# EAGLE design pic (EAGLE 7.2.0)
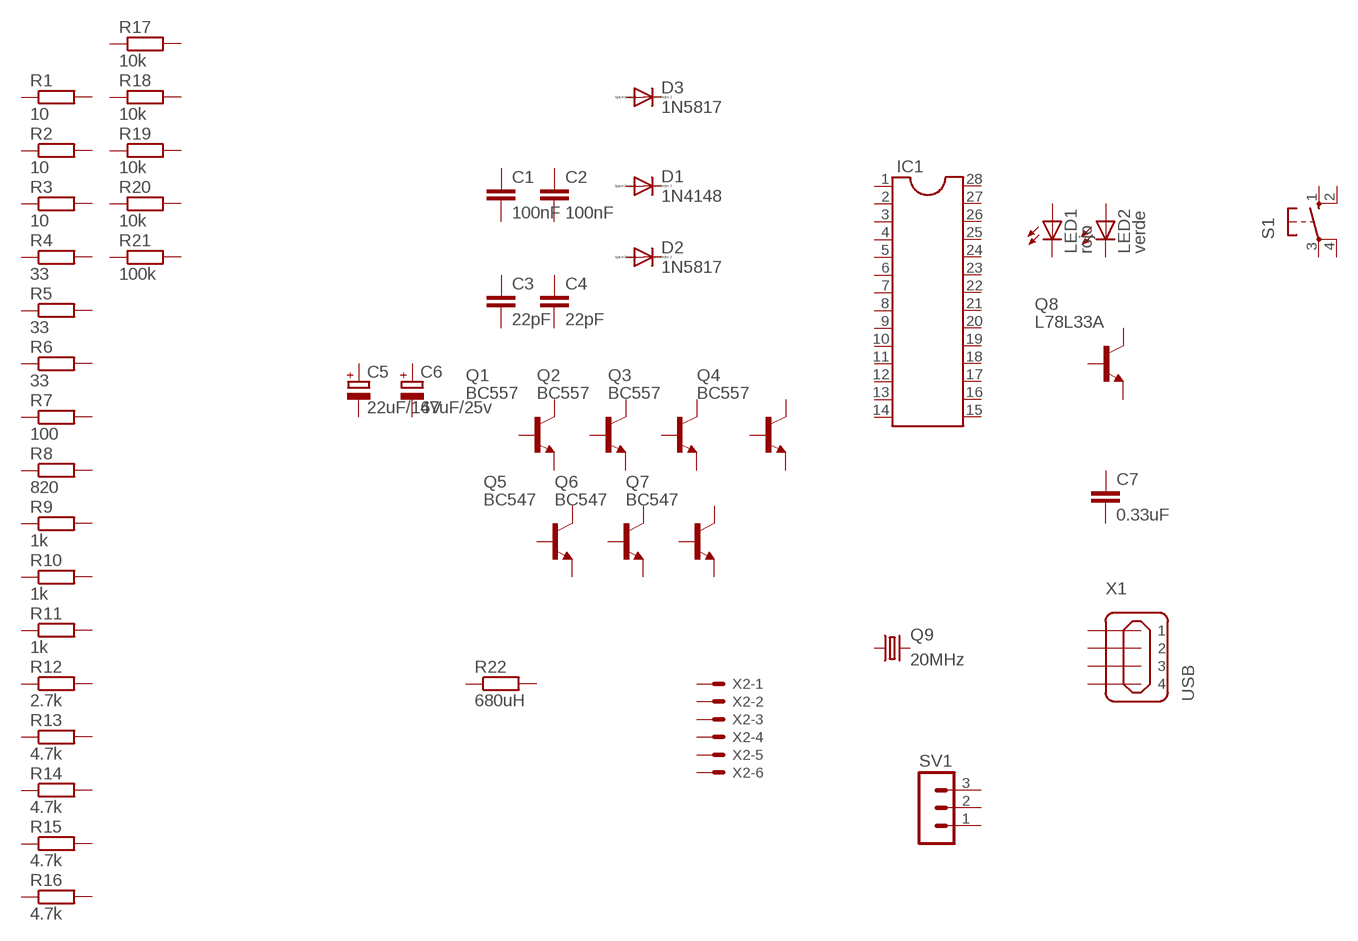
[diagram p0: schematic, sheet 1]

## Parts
C1  100nF  C-EU025-030X050  [C025-030X050]
C2  100nF  C-EU025-030X050  [C025-030X050]
C3  22pF  C-EU050-024X044  [C050-024X044]
C4  22pF  C-EU050-024X044  [C050-024X044]
C5  22uF/16V  CPOL-EUE2-5  [E2-5]
C6  47uF/25v  CPOL-EUE2-5  [E2-5]
C7  0.33uF  C-EU050-024X044  [C050-024X044]
D1  1N4148  1N4148DO35-7  [DO35-7]
D2  1N5817  1N4148DO35-7  [DO35-7]
D3  1N5817  1N4148DO35-7  [DO35-7]
IC1  DIL28-3  [DIL28-3]
LED1  rojo  LED3MM  [LED3MM]
LED2  verde  LED3MM  [LED3MM]
Q1  BC557  BCX59SMD  [TO92-EBC]
Q2  BC557  BCX59SMD  [TO92-EBC]
Q3  BC557  BCX59SMD  [TO92-EBC]
Q4  BC557  BCX59SMD  [TO92-EBC]
Q5  BC547  BCX59SMD  [TO92-EBC]
Q6  BC547  BCX59SMD  [TO92-EBC]
Q7  BC547  BCX59SMD  [TO92-EBC]
Q8  L78L33A  BC449  [TO92-EBC]
Q9  20MHz  CRYSTALHC49S  [HC49/S]
R1  10  R-EU_0207/7  [0207/7]
R2  10  R-EU_0207/7  [0207/7]
R3  10  R-EU_0207/7  [0207/7]
R4  33  R-EU_0207/7  [0207/7]
R5  33  R-EU_0207/7  [0207/7]
R6  33  R-EU_0207/7  [0207/7]
R7  100  R-EU_0207/7  [0207/7]
R8  820  R-EU_0207/7  [0207/7]
R9  1k  R-EU_0207/7  [0207/7]
R10  1k  R-EU_0207/7  [0207/7]
R11  1k  R-EU_0207/7  [0207/7]
R12  2.7k  R-EU_0207/7  [0207/7]
R13  4.7k  R-EU_0207/7  [0207/7]
R14  4.7k  R-EU_0207/7  [0207/7]
R15  4.7k  R-EU_0207/7  [0207/7]
R16  4.7k  R-EU_0207/7  [0207/7]
R17  10k  R-EU_0207/7  [0207/7]
R18  10k  R-EU_0207/7  [0207/7]
R19  10k  R-EU_0207/7  [0207/7]
R20  10k  R-EU_0207/7  [0207/7]
R21  100k  R-EU_0207/7  [0207/7]
R22  680uH  R-EU_0207/10  [0207/10]
S1  10-XX  [B3F-10XX]
SV1  MA03-1  [MA03-1]
X1  USB  MINI-USB_SHIELD4P-85-32004-00X  [85-32004-00X]
X2  22-23-2061  [22-23-2061]
Unconnected: C1.1 C1.2 C2.1 C2.2 C3.1 C3.2 C4.1 C4.2 C5.+ C5.- C6.+ C6.- C7.1 C7.2 D1.A D1.C D2.A D2.C D3.A D3.C IC1.1 IC1.2 IC1.3 IC1.4 IC1.5 IC1.6 IC1.7 IC1.8 IC1.9 IC1.10 IC1.11 IC1.12 IC1.13 IC1.14 IC1.15 IC1.16 IC1.17 IC1.18 IC1.19 IC1.20 IC1.21 IC1.22 IC1.23 IC1.24 IC1.25 IC1.26 IC1.27 IC1.28 LED1.A LED1.K(C) LED2.A LED2.K(C) Q1.B Q1.C Q1.E Q2.B Q2.C Q2.E Q3.B Q3.C Q3.E Q4.B Q4.C Q4.E Q5.B Q5.C Q5.E Q6.B Q6.C Q6.E Q7.B Q7.C Q7.E Q8.B Q8.C Q8.E Q9.1 Q9.2 R1.1 R1.2 R2.1 R2.2 R3.1 R3.2 R4.1 R4.2 R5.1 R5.2 R6.1 R6.2 R7.1 R7.2 R8.1 R8.2 R9.1 R9.2 R10.1 R10.2 R11.1 R11.2 R12.1 R12.2 R13.1 R13.2 R14.1 R14.2 R15.1 R15.2 R16.1 R16.2 R17.1 R17.2 R18.1 R18.2 R19.1 R19.2 R20.1 R20.2 R21.1 R21.2 R22.1 R22.2 S1.1(S) S1.2(S1) S1.3(P) S1.4(P1) SV1.1 SV1.2 SV1.3 X1.1 X1.2 X1.3 X1.4 X1.M1(S1) X1.M2(S2) X2.1 X2.2 X2.3 X2.4 X2.5 X2.6

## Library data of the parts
C1-C4 C7 = rcl:C-EU: CAPACITOR, European symbol
C5 C6 = rcl:CPOL-EU: POLARIZED CAPACITOR, European symbol
D1-D3 = diode:1N4148: DIODE
IC1 = ic-package:DIL28: Dual In Line
LED1 LED2 = led:LED: LED
Q1-Q7 = transistor-npn:BCX59*: NPN Transistor
Q8 = transistor-npn:BC449*: NPN Transistor
Q9 = crystal:CRYSTAL: CRYSTAL; OC_FARNELL: 1667008; OC_NEWARK: unknown
R1-R22 = rcl:R-EU_: RESISTOR, European symbol
S1 = switch-omron:10-XX: OMRON SWITCH; MPN: B3F-1000; OC_FARNELL: 176432; OC_NEWARK: 36M3542
SV1 = con-lstb:MA03-1: PIN HEADER; OC_FARNELL: unknown; OC_NEWARK: unknown
X1 = con-cypressindustries:MINI-USB_SHIELD4P-: MINI USB 4 Pol. Source: www.cypressindustries.com; OC_FARNELL: unknown; OC_NEWARK: unknown
X2 = con-molex:22-23-2061: .100" (2.54mm) Center Header - 6 Pin; MF: MOLEX; MPN: 22-23-2061; OC_FARNELL: 1462922; OC_NEWARK: 27C1933

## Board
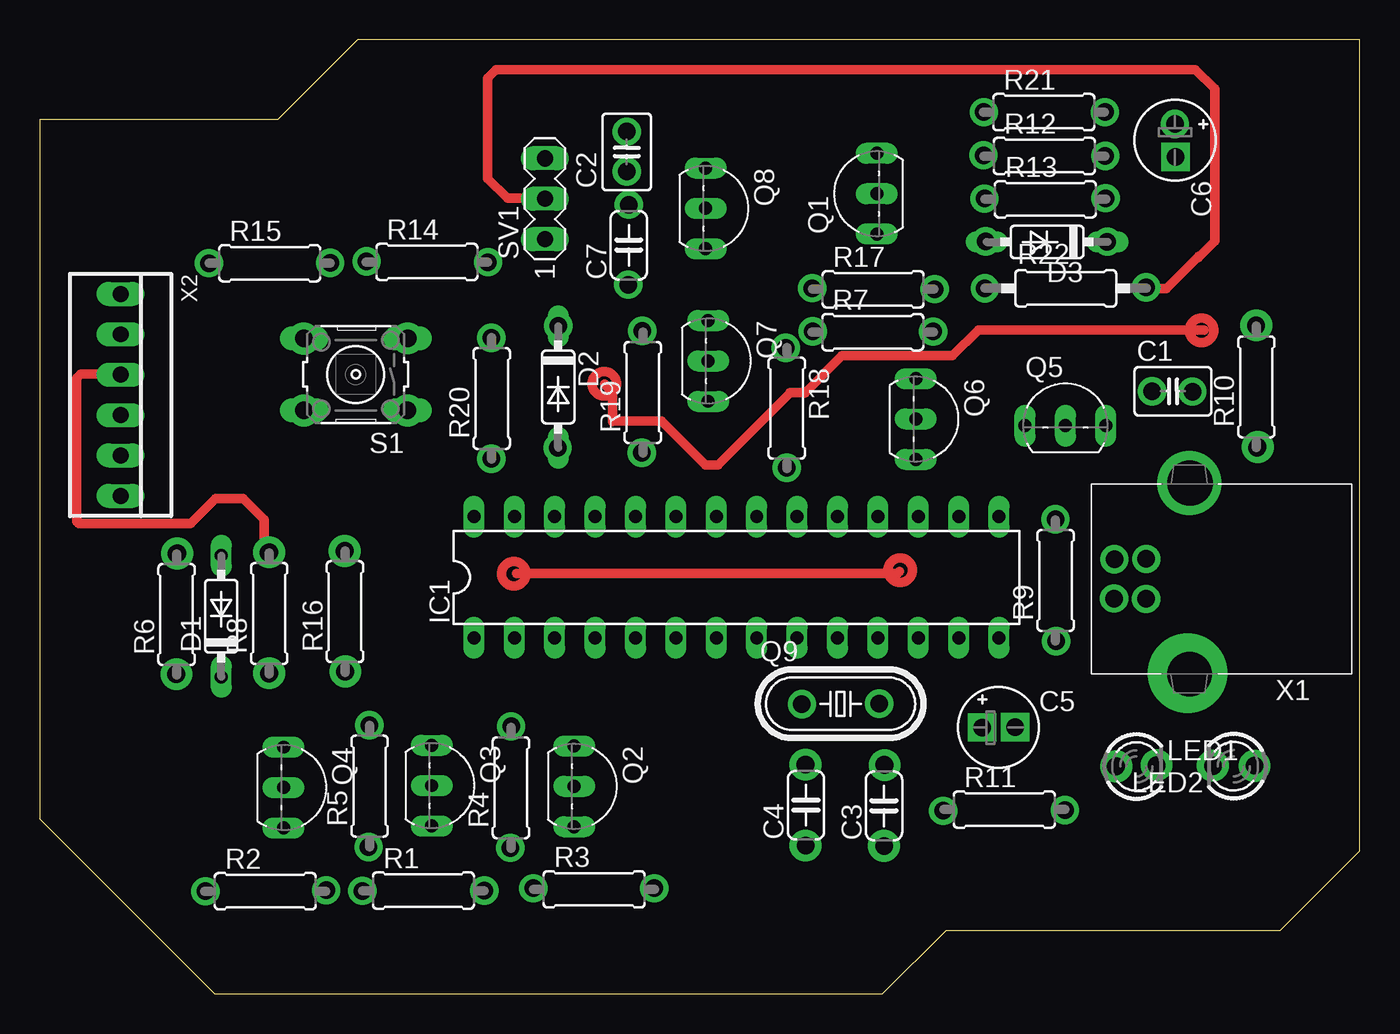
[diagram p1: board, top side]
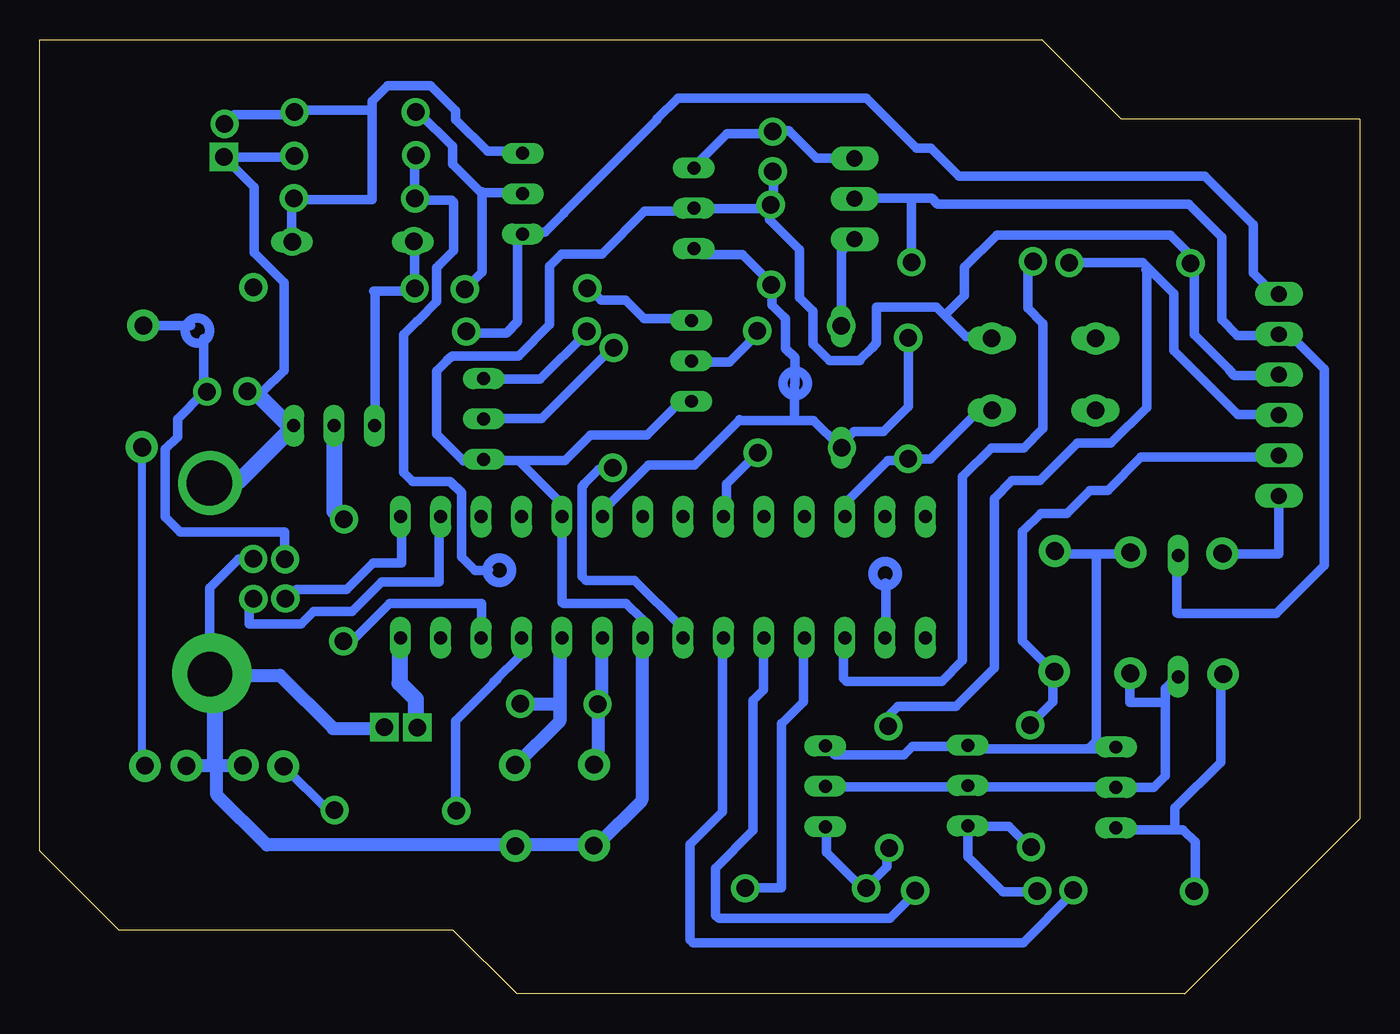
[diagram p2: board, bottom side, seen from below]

Size 83 x 60 mm. Coordinates in mm from the lower left corner, seen from the top.
Outline: 83,60 20,60 15,55 0,55 0,30 0,11 11,0 53,0 57,4 78,4 83,9 83,60
Copper layers (1*16): Top 0.035mm / dielectric 1.5mm / Bottom 0.035mm
Design rules "default": minimum track width 10mil, minimum drill 24mil, track to track 8mil, track to pad 8mil, pad to pad 8mil, via to via 8mil, smd to smd 8mil, copper to edge 40mil, drill to drill 8mil, minimum pad ring 10mil, minimum via ring 8mil, stop-mask expansion 4mil, vias tented up to drill 0mil, thermal gap 10mil

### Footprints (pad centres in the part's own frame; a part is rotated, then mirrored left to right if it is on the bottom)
C025-030X050 = drill 0.813 octagon: 1 -1.27,0; 2 1.27,0
C050-024X044 = drill 0.813 octagon: 1 -2.54,0; 2 2.54,0
E2-5 = drill 0.813 pad 1.27: + -1.016,0 | drill 0.813 pad 1.27 octagon: - 1.016,0
DO35-7 = drill 0.813 long: A 3.81,0; C -3.81,0
DIL28-3 = drill 0.813 long: 1 -16.51,-3.81; 2 -13.97,-3.81; 3 -11.43,-3.81; 4 -8.89,-3.81; 5 -6.35,-3.81; 6 -3.81,-3.81; 7 -1.27,-3.81; 8 1.27,-3.81; 9 3.81,-3.81; 10 6.35,-3.81; 11 8.89,-3.81; 12 11.43,-3.81; 13 13.97,-3.81; 14 16.51,-3.81; 15 16.51,3.81; 16 13.97,3.81; 17 11.43,3.81; 18 8.89,3.81; 19 6.35,3.81; 20 3.81,3.81; 21 1.27,3.81; 22 -1.27,3.81; 23 -3.81,3.81; 24 -6.35,3.81; 25 -8.89,3.81; 26 -11.43,3.81; 27 -13.97,3.81; 28 -16.51,3.81
LED3MM = drill 0.813 octagon: A -1.27,0; K 1.27,0
TO92-EBC = drill 0.813 long: B 0,-1.27; C -2.54,-1.27; E 2.54,-1.27
HC49/S = drill 0.813: 1 -2.413,0; 2 2.413,0
0207/7 = drill 0.813 octagon: 1 -3.81,0; 2 3.81,0
0207/10 = drill 0.813 octagon: 1 -5.08,0; 2 5.08,0
B3F-10XX = drill 1.016 long: 1 -3.251,2.261; 2 3.251,2.261; 3 -3.251,-2.261; 4 3.251,-2.261
MA03-1 = drill 1.016 long: 1 -2.54,0; 2 0,0; 3 2.54,0
85-32004-00X = drill 0.92 pad 1.27: 1 4.71,-1.25; 2 4.71,1.25; 3 2.71,1.25; 4 2.71,-1.25 | drill 2.3 pad 3: M1 0,6.02; M2 0,-6.02
22-23-2061 = drill 1 long: 1 -6.35,0; 2 -3.81,0; 3 -1.27,0; 4 1.27,0; 5 3.81,0; 6 6.35,0

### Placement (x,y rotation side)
C1  71.25,37.89 0 top
C2  36.91,52.95 90 top
C3  53.09,11.82 90 top
C4  48.17,11.86 90 top
C5  60.28,16.75 0 top
C6  71.39,53.68 270 top
C7  37.04,47.08 90 top
D1  11.41,23.75 90 top
D2  32.6,38.16 270 top
D3  63.34,47.29 180 top
IC1  43.81,26.2 0 top
LED1  68.95,14.3 0 top
LED2  75.08,14.31 180 top
Q1  51.37,50.32 90 top
Q2  34.88,13.05 270 top
Q3  25.91,13.1 270 top
Q4  16.6,12.97 270 top
Q5  64.5,37 0 top
Q6  56.35,36.15 270 top
Q7  43.29,39.8 270 top
Q8  43.14,49.4 270 top
Q9  50.35,18.24 0 top
R1  24.12,6.49 0 top
R2  14.18,6.46 0 top
R3  34.86,6.57 0 top
R4  29.63,12.96 90 top
R5  20.74,13.06 90 top
R6  8.6,23.85 90 top
R7  52.38,41.61 0 top
R8  14.43,23.92 90 top
R9  63.87,26 90 top
R10  76.5,38.17 90 top
R11  60.65,11.59 0 top
R12  63.16,52.69 0 top
R13  63.23,49.97 0 top
R14  24.34,46.03 0 top
R15  14.46,45.95 0 top
R16  19.19,24.04 90 top
R17  52.4,44.31 0 top
R18  46.97,36.84 270 top
R19  37.92,37.82 90 top
R20  28.42,37.45 90 top
R21  63.13,55.45 0 top
R22  64.51,44.37 0 top
S1  19.88,38.95 180 top
SV1  31.76,50 90 top
X1  72.28,26.09 180 top
X2  5.08,37.66 270 top

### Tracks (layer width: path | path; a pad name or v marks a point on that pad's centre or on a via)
N$1  (via drill 1.1 pad 1.78)
  other vias: 67.58,27.32
N$2  (via drill 1.1 pad 1.78)
  other vias: 69.58,27.35
N$3  (via drill 1.1 pad 1.78)
  other vias: 67.55,24.86
N$4  (via drill 1.1 pad 1.78)
  other vias: 69.56,24.84
N$5  (via drill 2.8 pad 3.81)
  other vias: 72.35,32.1
N$6  (via drill 2.8 pad 4)
  other vias: 72.3,20.11
N$7  (via drill 2.8 pad 4)
  other vias: 72.29,32.12
N$8
  Bottom 0.5: 76.59,34.34 76.59,14.53 76.42,14.36
N$9
  Bottom 0.61: 69.69,27.34 70.5,27.34 72.33,25.51 72.33,21.51 72.35,21.49
N$10
  Bottom 0.813: 72.15,20.02 67.9,20.02 64.56,16.69 61.42,16.69 61.33,16.79
N$11
  Bottom 0.813: 70.38,14.34 73.64,14.34 73.66,14.31
N$12
  Bottom 0.813: 72.08,14.36 72.08,19.99 72.12,20.04
N$13
  Bottom 0.5: 59.26,16.8 59.26,18.51 60.48,19.73 60.48,22.21 60.42,22.26
N$14
  Bottom 0.61: 64.46,11.53 64.86,11.53 67.59,14.25
N$15
  Bottom 0.61: 67.59,27.34 67.59,29.04 74.16,29.04 75.1,29.98 75.1,34.26 74.34,35.02 74.34,36.15 72.69,37.8 72.69,41.21
N$16
  Bottom 0.61: 76.42,42.09 76.38,42.04 73.51,42.04
N$17
  Bottom 0.61: 56.85,11.54 56.85,17.18 54.24,19.79
N$18
  Bottom 0.61: 47.61,22.31 47.61,18.66 47.88,18.4 47.88,14.7 48.11,14.46
N$19
  Bottom 0.61: 50.15,22.4 50.15,17.24 53.05,14.34
N$20
  Bottom 0.61: 52.7,18.19 50.34,18.19 50.31,18.21
N$21  (via drill 1.1 pad 1.78)
  other vias: 52.77,18.25
N$22  (via drill 1.1 pad 1.78)
  other vias: 47.92,18.21
N$23  (via drill 1.1 pad 1.78)
  other vias: 48.16,14.41
N$24  (via drill 1.1 pad 1.78)
  other vias: 53.11,14.4
N$25  (via drill 1.1 pad 1.78)
  other vias: 48.16,9.34
N$26  (via drill 1.1 pad 1.78)
  other vias: 53.11,9.3
N$27
  Bottom 0.61: 52.73,22.3 52.74,22.31
N$28
  Bottom 0.61: 52.71,22.3 52.71,21.34 54.45,19.6
N$29
  Bottom 0.61: 48.19,9.29 52.95,9.29 52.98,9.31 68.69,9.31 71.95,12.57 71.95,14.3 72.04,14.39
N$30
  Bottom 0.61: 61.92,35.81 61.92,44.11 62,44.19 59.62,44.19 59.42,44.39 59.42,47.25
N$31
  Bottom 0.61: 63.92,22.21 63.31,22.21 60.99,24.54 55.23,24.54 55.21,24.52 | 55.21,22.44 55.21,24.52 | 55.21,24.52 55.21,24.54
N$32
  Bottom 0.61: 57.89,29.98 57.89,25.89 61.51,25.89 63.36,24.04 65.78,24.04 66.56,23.25 69.8,23.25 69.83,23.27 69.83,24.52 69.6,24.75
N$33
  Bottom 0.61: 60.24,29.89 60.24,27.1 62.02,27.1 63.7,25.43 66.85,25.43 67.44,24.84
N$34
  Bottom 0.61: 64.58,35.54 64.58,30.56 63.92,29.91
N$35
  Bottom 0.61: 72.24,32.27 70.44,32.27 67.12,35.59
N$36
  Bottom 0.61: 69.85,37.77 69.14,37.77 67.1,35.74
N$37
  Bottom 1.016: 72.01,32.24 70.46,32.24 67.25,35.45 67.25,35.65 69.41,37.81
N$38
  Bottom 1.016: 64.49,35.49 64.49,30.36 63.92,29.8
N$39
  Bottom 1.016: 60.38,22.23 60.38,19.55 59.36,18.54 59.36,17.06 59.21,16.91
N$40
  Bottom 0.61: 67.15,47.09 67.15,49.83 67.06,49.91
N$41
  Bottom 0.61: 59.42,49.99 59.42,52.49 59.35,52.56
N$42
  Bottom 0.61: 71.4,52.61 67.16,52.61 67.11,52.56
N$43
  Bottom 0.61: 67.06,55.3 70.79,55.3 71.35,54.74
N$44
  Bottom 0.61: 69.96,37.9 68.94,37.9 67.64,39.2 67.64,44.73 69.51,46.6 69.51,50.73 71.35,52.56
N$45
  Bottom 0.61: 54.94,38.65 51.54,38.65 48.66,41.52
N$46
  Bottom 0.61: 54.77,26.66 54.83,26.61 55.62,26.61 56.49,27.48 56.49,31.51 57.19,32.21 59.55,32.21 60.12,32.79 60.12,41.45 59.26,42.31
N$47
  Bottom 0.61: 59.42,49.92 57.11,49.92 56.98,49.79 56.98,46.75 57.89,45.84 57.89,45.83 58.04,45.67 58.04,43.52 59.23,42.34
N$48  (via drill 1.1 pad 1.78)
  other vias: 59.42,44.36
N$49
  Bottom 0.61: 52.81,50.38 55.26,50.38 57.05,52.16 57.05,53.3 59.17,55.42
N$50
  Bottom 0.61: 55.2,50.44 55.2,45.4 56.24,44.36
N$51
  Bottom 0.61: 56.24,41.55 53.66,41.55 52.95,42.26 52.95,47.45 52.69,47.71
N$52
  Bottom 0.61: 52.77,52.99 54.85,52.99 56.84,54.98 56.84,55.54 58.42,57.12 61.12,57.12 62.11,56.14 62.11,49.95 67.01,49.95
N$53
  Bottom 0.61: 62.16,55.56 66.66,55.56 66.74,55.49
N$54
  Bottom 0.61: 42.27,42.48 45.01,42.48 46.17,43.64 47.7,43.64 48.45,44.39
N$55
  Bottom 0.61: 45.14,22.39 45.14,23.56 46.12,24.55 50.08,24.55 50.15,24.62 50.15,29.9 50.15,29.99 50.15,30.81 52.89,33.55 54.95,33.55 55,33.6
N$56
  Bottom 0.61: 54.96,36.19 51.44,36.19 47.1,40.52
N$57
  Bottom 0.61: 46.98,32.98 47.86,32.98 48.79,32.05 48.79,32.02 48.84,31.98 48.84,31.96 48.89,31.91 48.89,26.25 48.64,26 45.6,26 42.73,23.12
N$58
  Bottom 0.813: 47.69,22.38 47.69,18.41 47.9,18.2 47.9,14.69 48.11,14.47
N$59
  Bottom 0.61: 53.04,33.54 49.98,33.54 48.36,35.15 44.81,35.15 42.75,37.21
N$60
  Bottom 0.61: 36.88,51.67 36.88,49.84 37.02,49.69
N$61
  Bottom 0.61: 41.94,49.39 37.36,49.39 37.16,49.59
N$62
  Bottom 0.61: 37.04,54.1 39.77,54.1 41.91,51.96
N$63
  Bottom 0.61: 37.16,44.52 37.16,44.83 38.83,46.49 41.41,46.49 41.74,46.81
N$64
  Bottom 0.61: 55.21,33.5 56.35,33.5 58.05,35.2 58.05,39.15 57.38,39.83 57.38,39.85 57.27,39.95 57.26,39.95 57.2,40.01 57.17,40.01 57.08,40.11 52.9,40.11 50.94,42.08 50.94,45.76 50.17,46.52 47.65,46.52 44.96,49.21 42.26,49.21 42.14,49.34
N$65
  Bottom 0.61: 41.85,39.74 39.62,39.74 37.96,41.4
N$66
  Bottom 0.61: 39.83,30.11 39.83,32.06 37.94,33.95
N$67
  Bottom 0.61: 37.04,54.27 35.9,54.27 34.16,52.54 31.76,52.54 31.74,52.51
N$68
  Bottom 0.61: 47.5,30.91 47.08,30.91 44.73,33.26 41.83,33.26 39.02,36.06 | 39.02,36.06 38.99,36.1 | 39.02,36.06 34.34,36.06 32.71,34.44
N$69
  Bottom 0.61: 37.12,49.49 37.12,48.69 35.23,46.79 35.23,43.77 34.39,42.94 34.39,40.86 33.35,39.83 31.48,39.83 | 31.48,39.83 31.41,39.83 | 31.48,39.83 30.56,40.74
N$70  (via drill 1.1 pad 1.78)
  other vias: 71.42,52.64
N$71
  Bottom 0.61: 32.6,42.06 32.6,46.71 31.99,47.33
N$72
  Bottom 0.61: 28.38,41.15 28.38,36.94 29.94,35.38 31.8,35.38 32.6,34.58
N$73
  Bottom 0.61: 28.55,33.54 29.66,33.54 32.42,30.77
N$74
  Bottom 0.61: 23.3,41.33 24.75,41.33 26.61,43.19 30.39,43.19 30.39,40.92 30.69,40.62
N$75
  Bottom 0.61: 28.38,33.64 27,33.64 23.85,36.79
N$76
  Bottom 0.61: 31.8,50.04 28.2,50.04 | 28.2,50.04 28.2,46.02 | 28.2,50.04 26.91,50.04 26.55,49.67 10.75,49.67 8.66,47.59
N$77
  Bottom 0.61: 32.45,22.46 32.45,19.84 32.26,19.65 26.29,19.65 24.98,20.96 24.98,32.52 23.16,34.34 21.11,34.34 19.91,35.54 19.91,42.15 20.88,43.11 20.88,45.69 20.64,45.92
N$78
  Bottom 0.61: 5.08,38.89 7.88,38.89 8.21,39.23 8.21,39.26 10.4,41.45 10.4,45.73 10.54,45.86
N$79
  Bottom 0.61: 5.3,36.44 7.67,36.44 11.7,40.46 11.7,44.02 13.65,45.98 18.14,45.98 18.18,45.94
N$80
  Bottom 0.61: 5.31,41.4 7.69,41.4 8.68,42.39 8.68,47.55
N$81
  Bottom 0.61: 52.64,47.91 51.23,47.91 50.04,49.1 50.04,49.14 44.19,54.99 44.19,55.02 42.88,56.34 31.01,56.34 27.86,53.19 26.96,53.19 25.2,51.42 9.75,51.42 6.7,48.38 6.7,45.33 5.36,43.99
N$82
  Bottom 0.61: 29.7,16.82 29.7,17.41 29.04,18.07 25.4,18.07 22.99,20.49 22.99,31.15 21.86,32.27 20.11,32.27 17.75,34.64 15.64,34.64 13.4,36.88 13.4,45.51 13.44,45.55
N$83
  Bottom 0.61: 33.64,13.01 15.44,13.01 15.35,12.93
N$84
  Bottom 0.61: 15.38,15.4 24.4,15.4 24.57,15.57 28.11,15.57 28.66,15.03 33,15.03 33.55,15.57
N$85
  Bottom 0.61: 29.74,9.07 29.74,7.97 31.07,6.64
N$86
  Bottom 0.61: 33.52,10.47 33.52,8.91 31.23,6.61
N$87
  Bottom 0.61: 24.62,10.53 22.06,10.53 20.79,9.25
N$88
  Bottom 0.61: 24.65,10.45 24.65,8.62 22.44,6.41 20.43,6.41 20.38,6.46
N$89
  Bottom 0.61: 10.34,6.44 10.34,9.55 11.11,10.32 15.15,10.32 15.21,10.39
N$90
  Bottom 0.61: 34.98,22.23 34.98,18.36 36.34,17 36.38,17 36.38,6.67 38.56,6.67 38.56,6.61
N$91
  Bottom 0.61: 37.49,22.24 37.49,19.1 38.14,18.45 38.14,10.28 40.51,7.9 40.51,4.95 40.3,4.74 29.55,4.74 27.94,6.35
N$92
  Bottom 0.61: 40.08,22.34 40.08,11.44 42.12,9.39 42.12,3.41 41.92,3.21 21.16,3.21 18.12,6.25
N$93
  Bottom 0.61: 10.69,46.06 10.69,46.49 11.93,47.73 22.82,47.73 24.86,45.69 24.86,43.91 26.06,42.71
N$94
  Bottom 0.61: 19.29,20.23 19.29,18.36 20.74,16.91
N$95
  Bottom 0.61: 14.4,27.66 18.96,27.66 19.12,27.82
N$96
  Bottom 0.61: 16.57,27.62 16.57,15.91 16.98,15.51
N$97
  Bottom 0.61: 5.28,33.75 13.75,33.75 15.84,31.66 16.98,31.66 18.43,30.21 20.06,30.21 21.21,29.06 21.21,22.2 19.41,20.4
N$98
  Bottom 0.61: 15.31,12.99 12.96,12.99 12.24,13.71 12.24,19.21 11.47,19.98
N$99
  Bottom 0.61: 12.34,18.31 14.45,18.31 14.45,19.94
N$100
  Bottom 0.61: 8.75,19.9 8.75,14.55 11.61,11.69 11.61,10.53 11.66,10.47
N$101
  Bottom 0.61: 8.5,27.66 5.1,27.66 5.1,31.23
N$102
  Bottom 0.61: 11.49,27.66 11.49,23.96 11.45,23.93 5.26,23.93 2.24,26.95 2.24,39.29 4.47,41.52
N$103
  Top 0.61: 4.9,38.96 2.56,38.96 2.33,38.73 2.33,29.7 2.45,29.57 9.49,29.57 11.05,31.14 12.8,31.14 14.11,29.82 14.11,28.16 14.35,27.93
N$104
  Bottom 0.61: 29.79,22.35 29.79,25.8 29.82,25.84
N$105
  Top 0.61: 29.99,26.45 53.92,26.45 54.05,26.57
N$106
  Top 0.61: 31.2,50.02 29.41,50.02 28.16,51.27 28.16,57.59 28.7,58.12 72.66,58.12 73.88,56.91 73.88,47.33 72.86,46.31
N$107
  Top 0.61: 69.62,44.35 70.85,44.35 72.89,46.39
N$108
  Top 0.61: 73.21,41.74 59.01,41.74 57.4,40.12 50.44,40.12 48.1,37.79
N$109
  Top 0.61: 36.12,36.06 36.09,36.02 39.1,36.02 41.86,33.26 42.65,33.26 47.21,37.83
N$110
  Top 0.61: 47.16,37.8 48.12,37.8
N$111
  Top 0.61: 36,36 36,37.86 35.52,38.34
N$112
  Bottom 0.61: 35.55,36.12 35.55,38.3 35.52,38.33 35.52,40 36.1,40.58 36.1,42.45 36.15,42.5 36.23,42.58 36.96,43.31 36.96,44.36 37.04,44.44
N$113  (via drill 1.1 pad 1.27)
  other vias: 36.91,54.24
N$114  (via drill 1.1 pad 1.78)
  other vias: 36.91,54.23
N$115  (via drill 1.1 pad 1.78)
  other vias: 36.91,51.73
N$116  (via drill 1.1 pad 1.78)
  other vias: 37.04,49.62
N$117  (via drill 1.1 pad 1.78)
  other vias: 37,44.6
N$118  (via drill 1.1 pad 1.78)
  other vias: 37.89,41.69
N$119  (via drill 1.1 pad 1.78)
  other vias: 37.86,34.02
N$120  (via drill 1.1 pad 1.78)
  other vias: 46.98,33.09
N$121  (via drill 1.1 pad 1.78)
  other vias: 46.91,40.62
N$122  (via drill 1.1 pad 1.78)
  other vias: 48.6,41.66
N$123  (via drill 1.1 pad 1.78)
  other vias: 48.58,44.38
N$124  (via drill 1.1 pad 1.78)
  other vias: 56.26,44.31
N$125  (via drill 1.1 pad 1.78)
  other vias: 56.17,41.65
N$126  (via drill 1.1 pad 1.78)
  other vias: 59.4,50.01
N$127  (via drill 1.1 pad 1.78)
  other vias: 59.34,52.74
N$128  (via drill 1.1 pad 1.78)
  other vias: 67,52.69
N$129  (via drill 1.1 pad 1.78)
  other vias: 67.01,50.04
N$130  (via drill 1.1 pad 1.78)
  other vias: 59.36,55.45
N$131  (via drill 1.1 pad 1.78)
  other vias: 66.97,55.45
N$132  (via drill 1.1 pad 1.78)
  other vias: 71.38,54.71
N$133  (via drill 1.1 pad 1.78)
  other vias: 76.47,42
N$134  (via drill 1.1 pad 1.78)
  other vias: 69.56,44.42
N$135  (via drill 1.1 pad 1.78)
  other vias: 76.55,34.35
N$136  (via drill 1.1 pad 1.78)
  other vias: 69.95,37.89
N$137  (via drill 1.1 pad 1.78)
  other vias: 72.47,37.88
N$138  (via drill 1.1 pad 1.78)
  other vias: 63.86,29.84
N$139  (via drill 1.1 pad 1.78)
  other vias: 63.9,22.18
N$140  (via drill 1.1 pad 1.78)
  other vias: 67.66,14.3
N$141  (via drill 1.1 pad 1.78)
  other vias: 70.24,14.36
N$142  (via drill 1.1 pad 1.78)
  other vias: 73.78,14.32
N$143  (via drill 1.1 pad 1.78)
  other vias: 76.4,14.36
N$144  (via drill 1.1 pad 1.78)
  other vias: 64.46,11.55
N$145  (via drill 1.1 pad 1.78)
  other vias: 56.81,11.51
N$146  (via drill 1.1 pad 1.78)
  other vias: 29.59,9.18
N$147  (via drill 1.1 pad 1.78)
  other vias: 31.04,6.64
N$148  (via drill 1.1 pad 1.78)
  other vias: 38.64,6.64
N$149  (via drill 1.1 pad 1.78)
  other vias: 27.95,6.5
N$150  (via drill 1.1 pad 1.78)
  other vias: 20.29,6.47
N$151  (via drill 1.1 pad 1.78)
  other vias: 20.68,9.24
N$152  (via drill 1.1 pad 1.78)
  other vias: 18.01,6.51
N$153  (via drill 1.1 pad 1.78)
  other vias: 10.41,6.45
N$154  (via drill 1.1 pad 1.78)
  other vias: 29.64,16.82
N$155  (via drill 1.1 pad 1.78)
  other vias: 20.73,16.9
N$156  (via drill 1.1 pad 1.78)
  other vias: 19.2,20.25
N$157  (via drill 1.1 pad 1.78)
  other vias: 14.4,20.12
N$158  (via drill 1.1 pad 1.78)
  other vias: 8.57,20.09
N$159  (via drill 1.1 pad 1.78)
  other vias: 19.2,27.86
N$160  (via drill 1.1 pad 1.78)
  other vias: 14.38,27.75
N$161  (via drill 1.1 pad 1.78)
  other vias: 8.6,27.69
N$162  (via drill 1.1 pad 1.78)
  other vias: 28.39,33.65
N$163  (via drill 1.1 pad 1.78)
  other vias: 28.39,41.26
N$164  (via drill 1.1 pad 1.78)
  other vias: 10.64,45.95
N$165  (via drill 1.1 pad 1.78)
  other vias: 18.26,45.96
N$166  (via drill 1.1 pad 1.78)
  other vias: 20.55,46.06
N$167  (via drill 1.1 pad 1.78)
  other vias: 28.19,46.01
N$168  (via drill 1.1 pad 1.78)
  other vias: 61.33,16.76
N$169  (via drill 1.1 pad 1.78)
  other vias: 59.25,16.75
N$170  (via drill 1.1 pad 1.78)
  other vias: 59.48,47.33
N$171  (via drill 1.1 pad 1.78)
  other vias: 67.12,47.3
N$172  (via drill 1.1 pad 1.78)
  other vias: 32.56,34.34
N$173  (via drill 1.1 pad 1.78)
  other vias: 32.61,42
N$174
  Bottom 0.813: 53.16,14.32 53.1,14.32 50.29,17.14 50.29,22.11 50.14,22.26
N$175
  Bottom 0.813: 50.41,18.2 52.62,18.2 52.65,18.23
N$176
  Bottom 0.813: 45.14,22.16 45.14,12.18 47.95,9.36 68.71,9.36 71.86,12.51 71.86,19.66 72.1,19.9
N$177  (via drill 1 pad 3.81)
  other vias: 72.29,20.14
N$178  (via drill 1 pad 5)
  other vias: 72.19,20.16
N$179  (via drill 1 pad 4)
  other vias: 72.29,32.1
N$180  (via drill 1.1 pad 2)
  other vias: 16.6,41.21
N$181  (via drill 1.1 pad 2)
  other vias: 16.61,36.69
N$182  (via drill 1.1 pad 2)
  other vias: 23.14,41.23
N$183  (via drill 1.1 pad 2)
  other vias: 23.12,36.69
N$184  (via drill 1.1 pad 2)
  other vias: 76.39,14.34
N$185  (via drill 1.1 pad 2)
  other vias: 73.76,14.35
N$186  (via drill 1.1 pad 2)
  other vias: 70.22,14.39
N$187  (via drill 1.1 pad 2)
  other vias: 67.69,14.31
N$188  (via drill 1.1 pad 2)
  other vias: 76.49,42.04
N$189  (via drill 1.1 pad 2)
  other vias: 76.59,34.39
N$190  (via drill 1.1 pad 2)
  other vias: 14.43,27.77
N$191  (via drill 1.1 pad 2)
  other vias: 19.16,27.85
N$192  (via drill 1.1 pad 2)
  other vias: 8.65,27.7
N$193  (via drill 1.1 pad 2)
  other vias: 14.43,20.16
N$194  (via drill 1.1 pad 2)
  other vias: 19.21,20.27
N$195  (via drill 1.1 pad 2)
  other vias: 8.6,20.1
N$196  (via drill 1.1 pad 2)
  other vias: 48.15,9.32
N$197  (via drill 1.1 pad 2)
  other vias: 53.09,9.3
N$198  (via drill 1.1 pad 2)
  other vias: 48.14,14.41
N$199  (via drill 1.1 pad 2)
  other vias: 53.12,14.39
(copper drawn outside any net)
  shapes: Bottom circle x4, Top circle x4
